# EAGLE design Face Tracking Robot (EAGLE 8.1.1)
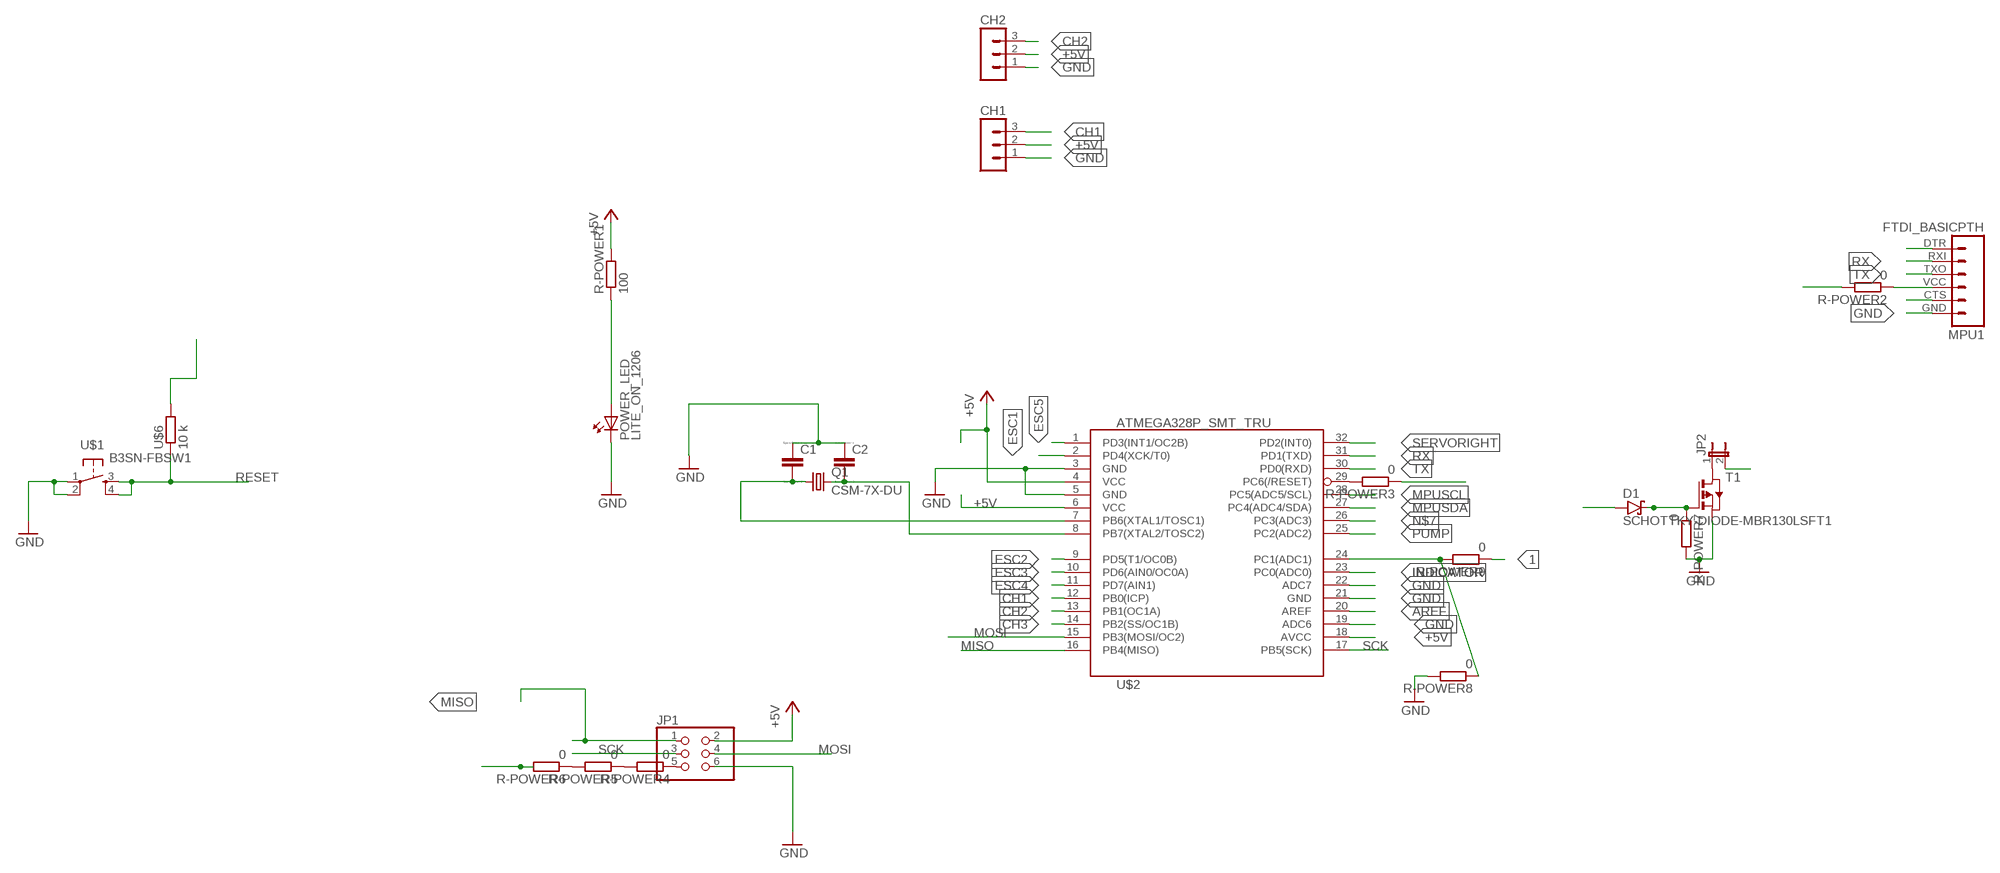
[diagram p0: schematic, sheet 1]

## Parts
C1  C  [C0805]
C2  C  [C0805]
CH1  MA03-1  [MA03-1]
CH2  MA03-1  [MA03-1]
D1  SCHOTTKY-DIODE-MBR130LSFT1  [SOD123FL]
JP1  PINHD-2X3-SMD  [2X03SMD]
JP2  JP1E  [JP1]
MPU1  FTDI_BASICPTH  [FTDI_BASIC]
POWER_LED  LITE_ON_1206  [1206]
Q1  CSM-7X-DU  [CSM-7X-DU]
R-POWER1  100  R_EUR_VISH  [R1206_VSHY]
R-POWER2  0  R_EUR_VISH  [R1206_VSHY]
R-POWER3  0  R_EUR_VISH  [R1206_VSHY]
R-POWER4  0  R_EUR_VISH  [R1206_VSHY]
R-POWER5  0  R_EUR_VISH  [R1206_VSHY]
R-POWER6  0  R_EUR_VISH  [R1206_VSHY]
R-POWER7  0  R_EUR_VISH  [R1206_VSHY]
R-POWER8  0  R_EUR_VISH  [R1206_VSHY]
R-POWER9  0  R_EUR_VISH  [R1206_VSHY]
T1  PMOSFETSOT23  [SOT-23]
U$1  B3SN-FBSW1  [B3SN-3112PAC-PL]
U$2  ATMEGA328P_SMT_TRU  [TQFP32-08-MILL_2]
U$6  10 k  R_EUR_VISH  [R1206_VSHY]

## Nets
1: MPU1.VCC R-POWER2.1 R-POWER9.1 U$6.2
+5V: CH1.2 CH2.2 JP1.2 JP2.2 R-POWER1.2 R-POWER2.2 U$2.4(VCC) U$2.6(VCC) U$2.18(AVCC)
AREF: U$2.20(AREF)
CH1: CH1.3 U$2.12(PB0(ICP))
CH2: CH2.3 U$2.13(PB1(OC1A))
CH3: U$2.14(PB2(SS/OC1B))
ESC1: U$2.2(PD4(XCK/T0))
ESC2: U$2.9(PD5(T1/OC0B))
ESC3: U$2.10(PD6(AIN0/OC0A))
ESC4: D1.A U$2.11(PD7(AIN1))
ESC5: U$2.1(PD3(INT1/OC2B))
G: D1.C R-POWER7.1 T1.3(G)
GND: C1.1 C2.1 CH1.1 CH2.1 JP1.6 MPU1.GND POWER_LED.C R-POWER7.2 R-POWER8.2 T1.2(S) U$1.1 U$1.2 U$2.3(GND) U$2.5(GND) U$2.19(ADC6) U$2.21(GND) U$2.22(ADC7)
INDICATOR: U$2.23(PC0(ADC0))
MISO: JP1.1 U$2.16(PB4(MISO))
MOSI: JP1.4 U$2.15(PB3(MOSI/OC2))
MPUSCL: U$2.28(PC5(ADC5/SCL))
MPUSDA: U$2.27(PC4(ADC4/SDA))
N$1: R-POWER8.1 R-POWER9.2 U$2.24(PC1(ADC1))
N$2: R-POWER3.2 U$2.29(PC6(/RESET))
N$3: JP1.5 R-POWER4.1
N$4: R-POWER4.2 R-POWER5.1
N$5: R-POWER5.2 R-POWER6.1
N$6: JP2.1 T1.1(D)
N$7: U$2.26(PC3(ADC3))
N$9: C2.2 Q1.2 U$2.8(PB7(XTAL2/TOSC2))
N$10: C1.2 Q1.1 U$2.7(PB6(XTAL1/TOSC1))
N$11: POWER_LED.A R-POWER1.1
N$21: MPU1.CTS
N$26: MPU1.DTR
PUMP: U$2.25(PC2(ADC2))
RESET: R-POWER3.1 R-POWER6.2 U$1.3 U$1.4 U$6.1
RX: MPU1.RXI U$2.31(PD1(TXD))
SCK: JP1.3 U$2.17(PB5(SCK))
SERVORIGHT: U$2.32(PD2(INT0))
TX: MPU1.TXO U$2.30(PD0(RXD))

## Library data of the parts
C1 C2 = eagle-ltspice:C: CAPACITOR, European symbol; SPICEMODEL: NONE; SPICEPREFIX: C
CH1 CH2 = con-lstb:MA03-1: PIN HEADER; OC_FARNELL: unknown; OC_NEWARK: unknown
D1 = bt_diode:SCHOTTKY-DIODE: Schottky Diode
JP1 = 1_206:PINHD-2X3-SMD: PIN HEADER
JP2 = jumper:JP1E: JUMPER
MPU1 = 1_206:FTDI_BASIC: FTDI Basic: 3.3V and 5V
POWER_LED = 1206:LITE_ON_1206: Luxeon K2 LED
Q1 = crystal:CSM-7X-DU: SMD CRYSTAL; OC_FARNELL: unknown; OC_NEWARK: unknown
R-POWER1-R-POWER9 U$6 = 1_206:R_EUR_VISH
T1 = fab:PMOSFET: MOS FET
U$1 = 1_206:B3SN-FBSW1
U$2 = 1_206:ATMEGA328P_SMT_TRU

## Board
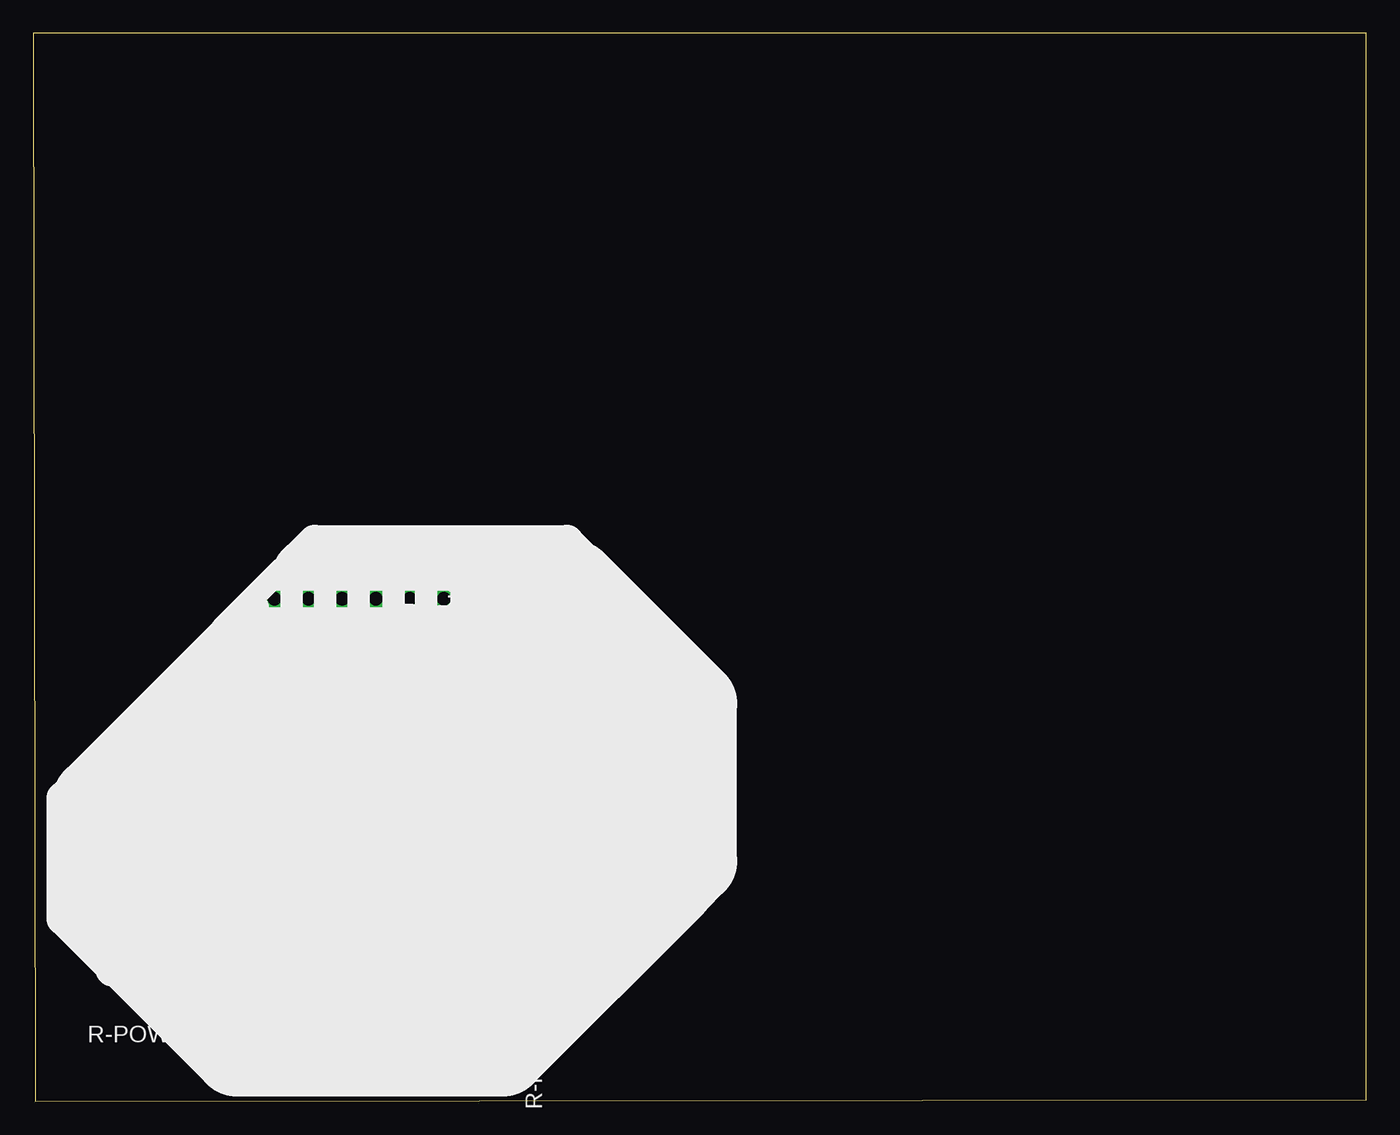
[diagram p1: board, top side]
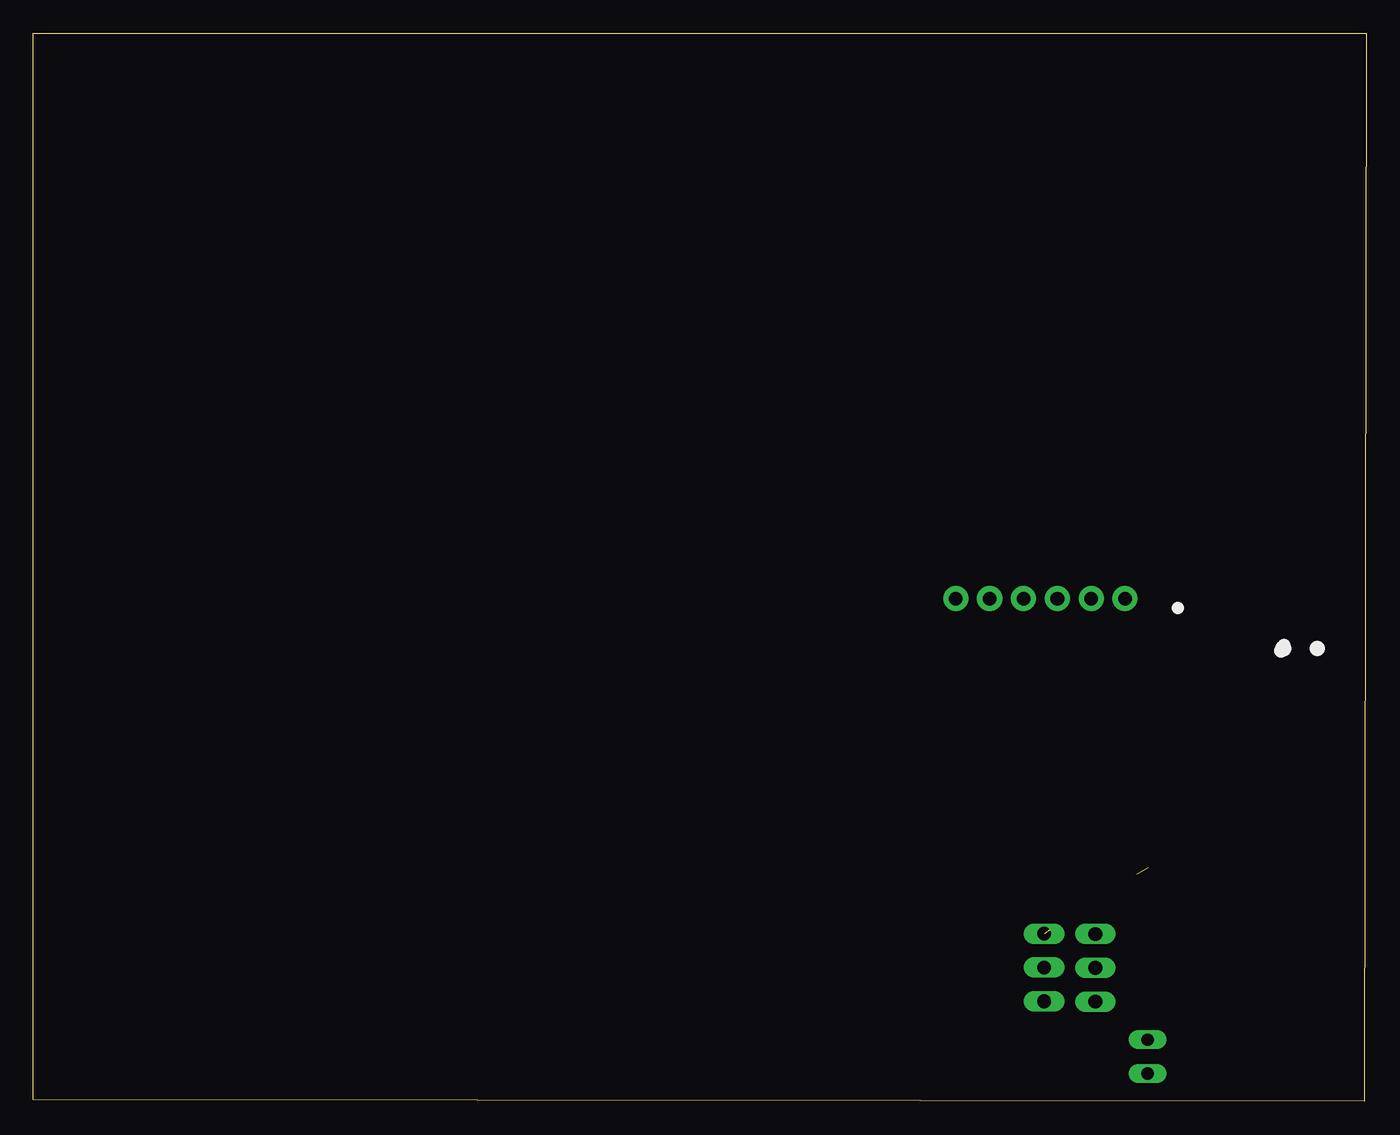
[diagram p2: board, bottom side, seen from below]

Size 100 x 80.13 mm. Coordinates in mm from the lower left corner, seen from the top.
Outline: 0.13,0 100,0.13 100,80.13 0,80.13 0.13,0
Copper layers (1*16): Top 0.035mm / dielectric 1.5mm / Bottom 0.035mm
Design rules "default": minimum track width 10mil, minimum drill 24mil, track to track 8mil, track to pad 8mil, pad to pad 8mil, via to via 8mil, smd to smd 8mil, copper to edge 40mil, drill to drill 8mil, minimum pad ring 10mil, minimum via ring 8mil, stop-mask expansion 4mil, vias tented up to drill 0mil, thermal gap 10mil

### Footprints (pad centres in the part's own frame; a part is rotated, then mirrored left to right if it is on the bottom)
C0805 = smd 1.3 x 1.5: 1 -0.95,0; 2 0.95,0
MA03-1 = drill 1.016 long: 1 -2.54,0; 2 0,0; 3 2.54,0
SOD123FL = smd 1.8 x 1.25: A 1.7,0; C -1.7,0
2X03SMD = smd 2.54 x 1.27: 1 -2.54,2.54; 2 2.92,2.54; 3 -2.54,0; 4 2.92,0; 5 -2.54,-2.54; 6 2.92,-2.54
JP1 = drill 0.914 long: 1 0,-1.27; 2 0,1.27
FTDI_BASIC = drill 1.016 pad 1.88: CTS 10.16,0; DTR 0,0; GND 12.7,0; RXI 2.54,0; TXO 5.08,0; VCC 7.62,0
1206 = smd 1.5 x 1.6: A -1.8,0; C 1.8,0
CSM-7X-DU = smd 5.5 x 2: 1 -4.75,0; 2 4.75,0
R1206_VSHY = smd 1.6 x 1.9: 1 -1.55,0; 2 1.55,0
SOT-23 = smd 0.787 x 0.889: 1 0.025,-1.016; 2 -0.94,1.016; 3 0.991,1.016
B3SN-3112PAC-PL = smd 2.75 x 1.4: 1 3.375,-2; 2 -3.375,-2; 3 3.375,2; 4 -3.375,2
TQFP32-08-MILL_2 = smd 1.65 x 0.392: 1 -4.293,2.8; 2 -4.293,2; 3 -4.293,1.2; 4 -4.293,0.4; 5 -4.293,-0.4; 6 -4.293,-1.2; 7 -4.293,-2; 8 -4.293,-2.8; 17 4.293,-2.8; 18 4.293,-2; 19 4.293,-1.2; 20 4.293,-0.4; 21 4.293,0.4; 22 4.293,1.2; 23 4.293,2; 24 4.293,2.8 | smd 0.392 x 1.65: 9 -2.8,-4.293; 10 -2,-4.293; 11 -1.2,-4.293; 12 -0.4,-4.293; 13 0.4,-4.293; 14 1.2,-4.293; 15 2,-4.293; 16 2.8,-4.293; 25 2.8,4.293; 26 2,4.293; 27 1.2,4.293; 28 0.4,4.293; 29 -0.4,4.293; 30 -1.2,4.293; 31 -2,4.293; 32 -2.8,4.293

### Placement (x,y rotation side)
C1  8.16,21.25 180 top
C2  15.37,21.33 0 top
CH1  20.32,10.01 90 top
CH2  24.16,10.04 90 top
D1  16.41,12.81 45 top
JP1  41.29,17.06 0 top
JP2  16.4,3.35 0 top
MPU1  18.09,37.72 0 top
POWER_LED  36.35,25.7 180 top
Q1  11.59,17.5 0 top
R-POWER1  43.02,25.22 0 top
R-POWER2  47.21,21.93 180 top
R-POWER3  30.67,33.87 180 top
R-POWER4  33.16,10.86 270 top
R-POWER5  35.79,7.71 270 top
R-POWER6  48.74,30.85 180 top
R-POWER7  12.37,6.8 180 top
R-POWER8  29.91,31.36 0 top
R-POWER9  25.96,34.03 270 top
T1  12.07,10.54 0 top
U$1  40.16,33.08 180 top
U$2  23.32,26.01 0 top
U$6  33.52,38.17 90 top

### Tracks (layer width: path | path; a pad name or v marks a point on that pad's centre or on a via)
1
  Top 0.406: R-POWER2.1 48.76,33.37 41.83,40.3 34.06,40.3 | 34.06,40.3 26.12,40.3 25.57,39.75 25.57,37.86 MPU1.VCC 25.96,37.47 R-POWER9.1 25.96,35.93 26.18,36.15 | 34.02,39.93 34.06,39.89 U$6.2 34.06,40.3
+5V
  Top 0.406: U$2.4 21.92,26.41 22.12,26.31 22.24,26.22 22.99,25.41 22.99,24.94 | 22.99,24.94 22.99,24.65 23.63,24.01 U$2.18 32.75,24.01 34,22.76 44.07,22.76 44.21,22.9 | U$2.6 21.1,24.8 21.24,24.94 22.99,24.94 | 44.17,19.6 JP1.2 | 44.21,21.92 44.21,22.9 | 44.21,21.92 JP1.2 | 44.21,22.9 44.21,24.86 R-POWER1.2 | JP1.2 45.93,19.6 46.29,19.24 46.29,16.23 46.21,16.15 46.21,16.13 45.89,15.81 42.51,15.81 41.94,15.24 41.94,12.61 39.66,10.79 24.45,10.79 CH2.2 | CH2.2 24.13,10.01 CH1.2 19.98,9.67 17.12,9.67 16.4,8.95 JP2.2 | CH2.2 25.21,10.04 25.28,10.11 | R-POWER2.2 44.22,21.93 44.21,21.92
CH1
  Top 0.406: U$2.12 22.92,21.7 22.99,17.71 20.42,15.14 CH1.3
CH2  (1 unrouted)
  Top 0.406: U$2.13 23.73,21.71 23.73,12.88
ESC4
  Top 0.406: U$2.11 22.12,18.77 22.05,18.7 22.05,18.09 19.42,15.46 18.82,15.46 17.61,14.26 D1.A
G
  Top 0.406: 13.29,11.82 13.29,11.77 13.08,11.56 T1.3 13.22,11.56 14.14,10.64 | 14.14,10.64 14.49,10.29 14.49,7.37 R-POWER7.1 | D1.C 15.12,11.61 14.14,10.64
GND
  Top 0.254: U$2.22 26.31,27.2 25.96,26.85 25.96,26.39 25.96,25.22 26.32,24.86 27.56,24.86 U$2.19 27.64,24.78 27.85,24.78
  Top 0.406: 18.43,25.61 U$2.5 17.39,25.61 16.75,26.25 | U$2.21 27.63,26.39 25.96,26.39 25.51,26.39 24.69,27.21 U$2.3 17.39,27.21 16.75,26.57 16.75,26.25 | C1.1 11.85,21.25 | 12.85,21.25 14.34,21.25 C2.1 | 28.33,27.19 28.31,27.21 U$2.22 29.09,27.21 29.16,27.14 | 29.16,27.14 29.16,29.35 30.48,30.63 30.48,31.35 | 30.48,31.35 30.47,36.99 MPU1.GND 31.15,38.23 35.82,38.23 36.78,37.36 U$1.1 U$1.2 | POWER_LED.C 30.61,25.7 30.26,26.04 | 30.26,26.04 29.16,27.14 | 30.26,26.04 31.94,27.72 45.3,27.72 47.29,25.86 47.16,25.73 47.16,20.32 47.64,19.84 47.64,15.64 46.52,14.52 JP1.6 45.75,14.52 38.73,7.5 CH2.1 24.13,7.47 CH1.1 | 16.75,26.25 16.69,26.19 7.4,26.19 3.18,21.97 3.18,15.74 4.56,14.36 9.64,14.36 9.91,14.64 | 9.91,14.64 12.13,16.85 12.13,20.97 11.85,21.25 | 11.85,21.25 12.85,21.25 | 12.85,21.25 12.87,21.23 | R-POWER8.2 30.49,31.36 30.48,31.35 | 9.91,14.64 11.13,13.42 T1.2 11,11.56 9.69,10.25 9.69,7.93 R-POWER7.2
  Top 0.61: CH2.1 24.32,7.34
MISO
  Top 0.406: JP1.1 28,19.6 26.39,21.21 26.39,21.45 U$2.16
MOSI
  Top 0.406: JP1.4 42.52,17.06 41.18,15.72 37.08,15.72 34.64,18.16 27.33,18.16 27.33,18.23 25.4,20.16 25.4,21.64 U$2.15
N$1
  Top 0.406: U$2.24 28.36,29.56 R-POWER8.1 27.08,31.36 R-POWER9.2
N$2
  Top 0.406: R-POWER3.2 24.25,33.87 22.93,32.55 22.93,30.31 U$2.29
N$3
  Top 0.406: R-POWER4.1 35.87,12.41 37.96,14.5 38.73,14.5 JP1.5
N$4
  Top 0.406: R-POWER5.1 33.21,9.26 R-POWER4.2
N$5
  Top 0.406: R-POWER6.1 50.29,16.59 41.55,7.85 41.55,7.84 40.23,6.52 36.15,6.52 R-POWER5.2
N$6
  Top 0.406: T1.1 12.1,8.5 12.41,8.18 12.41,4.79 12.39,4.77 12.52,4.77 15.22,2.07 15.75,2.07 15.76,2.08 JP2.1
N$9  (1 unrouted)
  Top 0.406: 18.78,23.1 18.92,23.1 U$2.8 17.19,23.21 17.19,21.33 | C2.2 17.19,21.33 | 17.19,21.33 17.19,17.01
N$10
  Top 0.406: Q1.1 6.84,17.72 6.19,17.72 6.19,17.33 6.11,17.33 6.11,21.25 C1.2 8.05,22.09 8.05,22.17 9.89,24.01 U$2.7
N$11
  Top 0.406: POWER_LED.A 40.99,25.7 R-POWER1.1
RESET
  Top 0.406: U$1.3 36.52,31.08 36.26,31.34 | 36.24,31.62 U$1.3 | U$1.3 U$1.4 46.96,31.08 R-POWER6.2 | 33.52,34.06 U$6.1 | 33.52,34.06 33.52,32.19 34.4,31.31 36.55,31.31 U$1.3 | R-POWER3.1 33.33,33.87 33.52,34.06
RX
  Top 0.406: U$2.31 21.32,37.03 MPU1.RXI
SCK
  Top 0.406: 38.41,17.22 38.57,17.06 JP1.3 39.41,17.06 41.51,19.16 41.51,21.1 41.62,21.21 29.61,21.21 U$2.17
TX
  Top 0.406: U$2.30 22.12,36.67 MPU1.TXO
